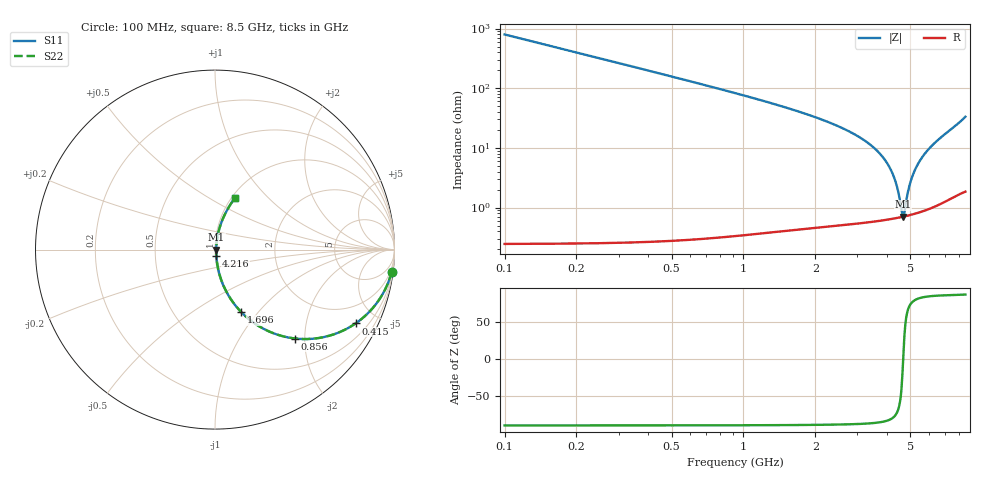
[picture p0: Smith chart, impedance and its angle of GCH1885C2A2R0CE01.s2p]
!Murata Part Number: GCH1885C2A2R0CE01
!These Parameters are Measured in Series Mode Connection
!Data Generated on Mar 13, 2026
!  o--ll--o
!Port1  Port2
!  o------o
!Operation Temp=25[degC], DC Bias Voltage=0[V]
!Freq. Start=100[MHz] Stop=9[GHz] 401[Steps]
# Hz S RI R 50
!Freq.(Hz) S11(Real) S11(Imag) S21(Real) S21(Imag) S12(Real) S12(Imag) S22(Real) S22(Imag)
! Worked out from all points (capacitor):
!   401 points, 100 MHz to 8.5 GHz, reference 50 ohm
!   read as one part in series: C = 2 pF near 142 MHz
!   lowest |Z| = 706 mohm at 4.657 GHz (marker M1)
!   series resonance near 4.666 GHz, so ESL is about 580 pH
!   S11 on the Smith chart (normalised r, x): 100 MHz: 1, -16; 415 MHz: 1.01, -3.80; 856 MHz: 1.01, -1.80; 1.696 GHz: 1.01, -0.82; 4.216 GHz: 1.01, -0.07; 8.5 GHz: 1.04, +0.67
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1e8  0.9844 -0.1238  0.0156 0.1238  0.0156 0.1238  0.9844 -0.1238
2.47e8  0.9115 -0.2836  0.0885 0.2836  0.0885 0.2836  0.9115 -0.2836
4.15e8  0.7832 -0.4114  0.2168 0.4114  0.2168 0.4114  0.7832 -0.4114
6.25e8  0.6098 -0.4866  0.3902 0.4866  0.3902 0.4866  0.6098 -0.4866
8.56e8  0.4471 -0.4954  0.5529 0.4954  0.5529 0.4954  0.4471 -0.4954
1.507e9  0.1859 -0.3847  0.8141 0.3847  0.8141 0.3847  0.1859 -0.3847
1.696e9  0.1459 -0.3479  0.8541 0.3479  0.8541 0.3479  0.1459 -0.3479
2.914e9  0.0328 -0.1632  0.9672 0.1632  0.9672 0.1632  0.0328 -0.1632
3.712e9  0.0124 -0.0799  0.9876 0.0799  0.9876 0.0799  0.0124 -0.0799
4.216e9  0.00775 -0.0357  0.9923 0.0357  0.9923 0.0357  0.00775 -0.0357
4.3e9  0.00739 -0.0288  0.9926 0.0288  0.9926 0.0288  0.00739 -0.0288
4.426e9  0.00705 -0.0187  0.993 0.0187  0.993 0.0187  0.00705 -0.0187
4.615e9  0.00694 -0.00389  0.9931 0.00389  0.9931 0.00389  0.00694 -0.00389
4.657e9  0.00698 -0.000659  0.993 0.000659  0.993 0.000659  0.00698 -0.000659
4.72e9  0.00708 0.00414  0.9929 -0.00414  0.9929 -0.00414  0.00708 0.00414
4.909e9  0.00767 0.0183  0.9923 -0.0183  0.9923 -0.0183  0.00767 0.0183
5.077e9  0.00853 0.0306  0.9915 -0.0306  0.9915 -0.0306  0.00853 0.0306
5.35e9  0.0106 0.05  0.9894 -0.05  0.9894 -0.05  0.0106 0.05
5.707e9  0.0144 0.0748  0.9856 -0.0748  0.9856 -0.0748  0.0144 0.0748
6.295e9  0.0236 0.1146  0.9764 -0.1146  0.9764 -0.1146  0.0236 0.1146
7.114e9  0.0433 0.1707  0.9567 -0.1707  0.9567 -0.1707  0.0433 0.1707
8.5e9  0.1127 0.2897  0.8873 -0.2897  0.8873 -0.2897  0.1127 0.2897
